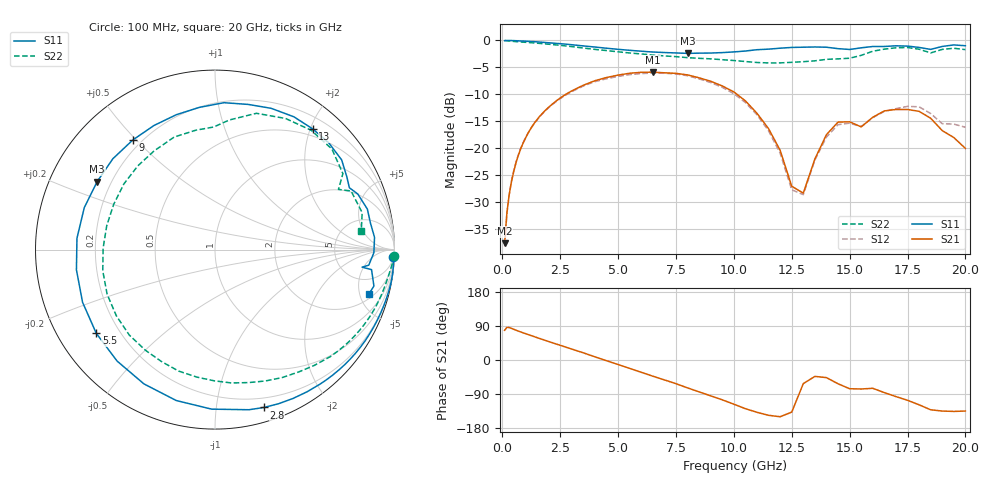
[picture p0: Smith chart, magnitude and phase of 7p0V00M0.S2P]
! Infineon Technologies  Discrete & RF Semiconductors
! bfp620
! VCE =  0.0 V,  IC =  0.0 mA
! Common Emitter S-Parameters:  Sep 2002
# GHz  S  MA  R  50
!  f  S11  S21  S12  S22
! GHz  MAG  ANG  MAG  ANG  MAG  ANG  MAG  ANG
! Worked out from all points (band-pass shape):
!   59 points, 100 MHz to 20 GHz, reference 50 ohm
!   highest |S21| = -5.90 dB at 6.5 GHz (marker M1); lowest = -37.7 dB at 100 MHz (marker M2)
!   |S21| within 3 dB of the highest: 3.234 GHz to 9.693 GHz (6.459 GHz wide, 99.9 % of centre)
!   lowest |S11| = -2.4 dB at 8 GHz (marker M3), VSWR 7.26, Z = 7.37 + j13.1 ohm
!   |S11| at or under -10 dB: nowhere
!   |S22| runs from -4.2 to 0.0 dB; largest |S21 - S12| = 0.059
!   S11 on the Smith chart (normalised r, x): 100 MHz: 6, -49; 2.8 GHz: 0.12, -1.35; 5.5 GHz: 0.12, -0.31; 9 GHz: 0.17, +0.49; 13 GHz: 0.38, +2.04; 20 GHz: 2.50, -6.07
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0.1  0.995 -2.3  0.013 78.4  0.0122 87.4  0.9995 -1.9
0.3  0.9986 -8.0  0.037 85.6  0.0371 84.7  0.9881 -5.3
0.8  0.9886 -20.9  0.099 73.9  0.0996 73.6  0.9673 -12.5
1.6  0.966 -41.6  0.195 57.0  0.1936 56.5  0.939 -23.7
2.8  0.9207 -72.8  0.321 32.8  0.3156 32.2  0.8858 -40.1
3.5  0.8891 -91.2  0.383 18.9  0.3772 18.3  0.8495 -49.5
5.5  0.8094 -144.8  0.495 -22.1  0.4811 -21.9  0.7643 -75.8
6.5  0.7802 -171.7  0.507 -42.7  0.4969 -41.9  0.731 -90.4
7  0.7717 175.3  0.5 -52.5  0.4949 -52.0  0.7176 -98.0
8  0.758 150.0  0.478 -73.6  0.4693 -73.6  0.6914 -115.5
9  0.7634 126.9  0.417 -94.6  0.4058 -94.6  0.6743 -135.1
10.5  0.7971 96.3  0.274 -128.5  0.2645 -127.8  0.6364 -169.3
11.5  0.8298 77.1  0.151 -146.0  0.1442 -145.1  0.6177 167.5
12.5  0.8606 59.3  0.044 -137.5  0.0408 -134.2  0.6258 144.2
13  0.8651 51.0  0.038 -62.3  0.0368 -57.3  0.6345 132.6
13.5  0.8692 43.2  0.079 -43.3  0.0771 -40.2  0.646 121.7
14.5  0.8386 28.8  0.174 -62.7  0.1646 -57.2  0.6737 99.2
15.5  0.8536 21.3  0.157 -76.5  0.158 -69.6  0.7265 83.7
16  0.8783 14.9  0.193 -74.7  0.1914 -67.9  0.7937 73.1
17  0.8914 4.4  0.228 -96.5  0.2319 -86.0  0.8539 51.1
18  0.861 -5.8  0.219 -118.2  0.2414 -107.9  0.8288 30.7
20  0.8924 -16.1  0.099 -134.7  0.1558 -126.8  0.8217 7.3
